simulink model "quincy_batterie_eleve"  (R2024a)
settings: Solver=FixedStepAuto  StartTime=0.0  StopTime=3600*4  RelTol=1e-3
libraries: fl_lib x4, nesl_utility x3, batteryecm_lib x1

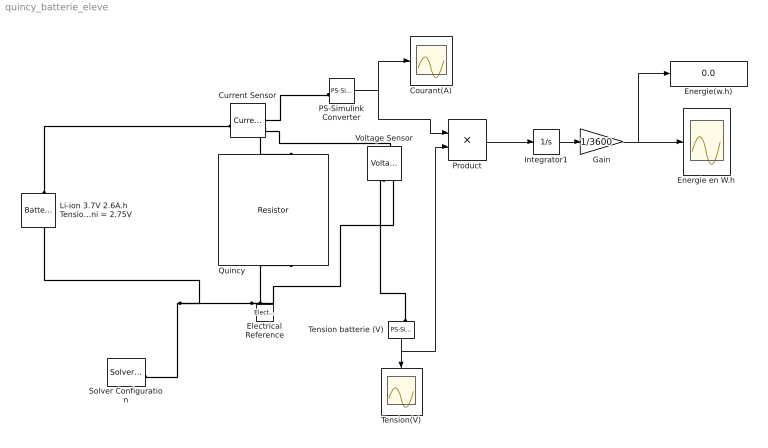
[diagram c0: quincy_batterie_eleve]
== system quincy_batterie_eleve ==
  Courant(A) : Scope
  Current Sensor : fl_lib/Electrical/Electrical Sensors/Current Sensor
  Electrical Reference : fl_lib/Electrical/Electrical Elements/Electrical Reference
  Energie en W.h : Scope
  Energie(w.h) : Display
  Gain : Gain  Gain=1/3600
  Integrator1 : Integrator
  Li-ion 3.7V 2.6A.h Tension mini = 2.75V : batteryecm_lib/Battery  Vnom=0 V  prm_dir=simscape.enum.battery.prm_dir.disabled  R1_dis=2 Ohm  R1_ch=2 Ohm  R1=0.065 Ohm  prm_AH=2  AH=0 hr*A  V1=2.8 V  AH1=0.8 hr*A  prm_R2=1  R2=2000 Ohm  Tmeas=298.15 K  charge_measurement_port=simscape.enum.battery.enable.no  prm_dyn=simscape.enum.battery.prm_dyn.off  Rp1=0.005 Ohm  tau1=30 s  Rp2=0.005 Ohm  tau2=30 s  Rp3=0.005 Ohm  tau3=30 s  Rp4=0.005 Ohm  tau4=30 s  Rp5=0.005 Ohm  tau5=30 s  prm_fade=1  N_fade=100  AH_fade=45 hr*A  R1_fade=2.02 Ohm  R1_ch_fade=2.02 Ohm  V1_fade=10.35 V  prm_age=simscape.enum.battery.prm_age.disabled  prm_age_OCV=simscape.enum.battery.prm_age_OCV.OCV  OCV_age=0.9  SOC_age=60  Tmeas_age=298.15 K  delta_time_age_vec=[0] d  temperature_age_vec=[273] K  OCV_scaling_age=2.2134e6  OCV_offset_age=1.632e6  temp_exp_age=0.515833569 V  t_exp_age=0.75  Vnom_T2=12 V  R1_T2=2.2 Ohm  R1_T2_dis=2.2 Ohm  R1_T2_ch=2.2 Ohm  V1_T2=11.4 V  R2_T2=2200 Ohm  Rp1_T2=0.005 Ohm  tau1_T2=30 s  Rp2_T2=0.005 Ohm  tau2_T2=30 s  Rp3_T2=0.005 Ohm  tau3_T2=30 s  Rp4_T2=0.005 Ohm  tau4_T2=30 s  Rp5_T2=0.005 Ohm  tau5_T2=30 s  Tmeas2=273.15 K  thermal_port=simscape.enum.thermaleffects.omit  thermal_mass=30000 J/K  i_specify=off  i_priority=None  i=0 A  i_nominal_specify=off  i_nominal_value=1  i_nominal_unit=A  v_specify=on  v_priority=Low  v=3 V  v_nominal_specify=off  v_nominal_value=1  v_nominal_unit=V  charge_specify=on  charge_priority=High  charge=2.6 hr*A  charge_nominal_specify=off  charge_nominal_value=1  charge_nominal_unit=hr*A  num_cycles_specify=off  num_cycles_priority=High  num_cycles=0  num_cycles_nominal_specify=off  num_cycles_nominal_value=1  num_cycles_nominal_unit=1  temperature_specify=off  temperature_priority=High  temperature=298.15 K  temperature_nominal_specify=off  temperature_nominal_value=1  temperature_nominal_unit=K
  PS-Simulink Converter : nesl_utility/PS-Simulink Converter  PhysicalDomain=network_engine_domain  SubClassName=ps_output  LeftPortType=input  RightPortType=output  PseudoPeriodic=off  Frequencies=[]  VectorFormat=1-D array  Unit=A  AffineConversion=off
  Product : Product  Inputs=**
  Quincy : fl_lib/Electrical/Electrical Elements/Resistor  R=3.94 Ohm  i_specify=off  i_priority=None  i=0 A  i_nominal_specify=off  i_nominal_value=1  i_nominal_unit=A  v_specify=off  v_priority=None  v=0 V  v_nominal_specify=off  v_nominal_value=1  v_nominal_unit=V
  Solver Configuration : nesl_utility/Solver Configuration  PhysicalDomain=network_engine_domain  SubClassName=solver  LeftPortType=input  RightPortType=generic  Tones=[]  Harmonics=[]  SimulateNoise=off  Profile=off  UseLocalSampling=off  EnableSwitchedLinearOptims=on  FrequencyDomain=off  UseCCode=off  RelTol=0.001  AbsTol=1e-06  MinStep=1e-09  ToWorkspace=off  RevertToSquareIcSolve=off  NumHomotopyIterations=100  PhasorMode=off  PhasorModeNumHarmonics=1  ConsistencySolver=NEWTON_FTOL  IndexReductionMethod=DerivativeReplacement  DoDC=off  ResidualTolerance=1e-09  ConsistencyTolSource=GLOBAL  ConsistencyAbsTol=0.001  ConsistencyRelTol=0.001  ConsistencyTolFactor=0.001  UseLocalSolver=off  LocalSolverChoice=NE_BACKWARD_EULER_ADVANCER  ResolveIndetEquations=on  FunctionEvalNumThread=1  LocalSolverSampleTime=0.001  DoFixedCost=off  MaxNonlinIter=3  MaxModeIter=2  ComputeImpulses=off  ImpulseIterations=2  LinearAlgebra=Sparse  LinearAlgebraNumThread=0  EquationFormulation=NE_TIME_EF  DelaysMemoryBudget=1024  AutomaticFiltering=on  FilteringTimeConstant=0.001  PartitionStorageMethod=AS_NEEDED  PartitionMemoryBudget=1024  PartitionMethod=FAST  MultibodyUseLocalSolver=off  MultibodyLocalSolverChoice=ODE1  MultibodyLocalSolverSampleTime=0.001
  Tension batterie (V) : nesl_utility/PS-Simulink Converter  PhysicalDomain=network_engine_domain  SubClassName=ps_output  LeftPortType=input  RightPortType=output  PseudoPeriodic=off  Frequencies=[]  VectorFormat=1-D array  Unit=V  AffineConversion=off
  Tension(V) : Scope
  Voltage Sensor : fl_lib/Electrical/Electrical Sensors/Voltage Sensor
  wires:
  PS-Simulink Converter/1 -> Product/1, Courant(A)/1
  Integrator1/1 -> Gain/1
  Gain/1 -> Energie(w.h)/1, Energie en W.h/1
  Product/1 -> Integrator1/1
  Tension batterie (V)/1 -> Product/2, Tension(V)/1
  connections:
  Solver Configuration/RConn1 -- Li-ion 3.7V 2.6A.h Tension mini = 2.75V/RConn1 -- Voltage Sensor/RConn2 -- Quincy/RConn1 -- Electrical Reference/LConn1
  Current Sensor/RConn2 -- Voltage Sensor/LConn1 -- Quincy/LConn1
  Current Sensor/RConn1 -- PS-Simulink Converter/LConn1
  Tension batterie (V)/LConn1 -- Voltage Sensor/RConn1
  Li-ion 3.7V 2.6A.h Tension mini = 2.75V/LConn1 -- Current Sensor/LConn1
